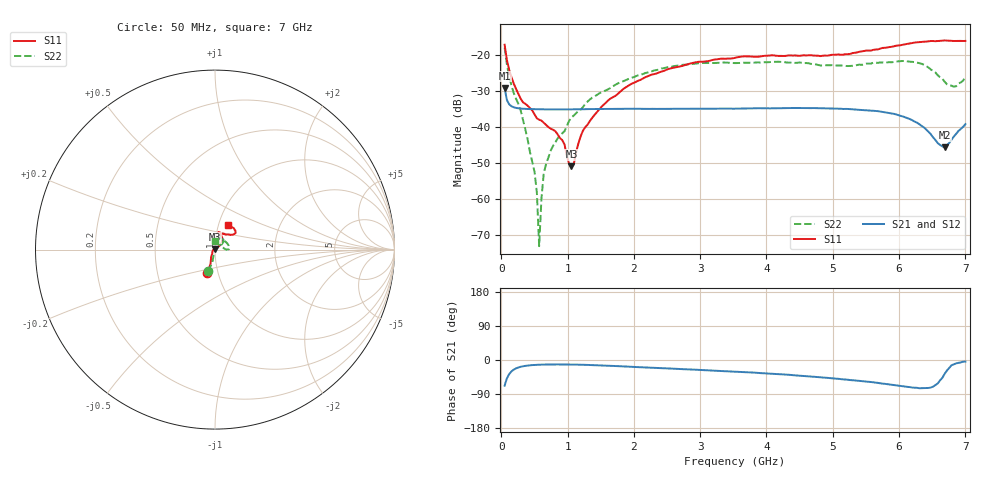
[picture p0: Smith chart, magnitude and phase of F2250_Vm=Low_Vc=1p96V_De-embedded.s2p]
! Integrated Device Technology
! Corporate Headquarters
! 6024 Silver Creek Valley Road
! San Jose, CA 95138  USA
! Phone:  1-408-284-8200
! Toll Free:  1-800-223-1366
! Webpage:  http://www.idt.com/
! Timing and RF Division
! 515 Groton Road, Suite 102
! Westford, MA 01886-6024
! Device:  F2250
! Description: Voltage Variable RF Attenuator
! Frequency:  50.0 -  6000.00 MHz
! Package:  3x3 mm Thin QFN Plastic Package: 16 pin
! Ports:  2 RF, 3 DC
!  Pin  1  = GND
!  Pin  2  = NC
!  Pin  3  = RF1  = Port 1
!  Pin  4  = NC
!  Pin  5  = GND
!  Pin  6  = GND
!  Pin  7  = GND
!  Pin  8  = GND
!  Pin  9  = NC
!  Pin 10  = RF2  = Port 2
!  Pin 11  = NC
!  Pin 12  = GND
!  Pin 13  = GND
!  Pin 14  = VCNTRL
!  Pin 15  = VDD
!  Pin 16  = VMODE
! Vcntrl:  1.960 Volts
! Vmode:  +0.000 Volts
! Vdd:  +3.30  Volts
! Current:  1.182 mA
! Data:  The device was measured on a the F2250 evaluation board which has
!  individual transmission lines to the RF pins.  Data was collected
!  using a calibrated network analyzer.  The evaluation board was
!  de-embedded using a TRL calibration technique.
!  The reference plane is the edge of the package pin.
! Misc:  SN 10
!  Action Tracker AT0258
! Date Measured:  2014-11-26
! Date:  2015-10-15  MJV
! Note:
!  Integrated Device Technology supplies this data as a sample of measured
!  data at the package pin for this product.  Your particular data for this
!  product may vary.
!  Data was taken at 25 degrees C.
!  Integrated Device Technology reserves the right to change this data at anytime.
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# GHz S dB R 50
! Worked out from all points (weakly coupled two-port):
!   201 points, 50 MHz to 7 GHz, reference 50 ohm
!   highest |S21| = -29.22 dB at 50 MHz (marker M1); lowest = -45.7 dB at 6.687 GHz (marker M2)
!   lowest |S11| = -51.0 dB at 1.058 GHz (marker M3), VSWR 1.01, Z = 49.9 + j0.24 ohm
!   |S11| at or under -10 dB: start of sweep to end of sweep
!   |S22| runs from -73.1 to -18.0 dB; largest |S21 - S12| = 5.4e-05
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0.05  -17.18 -108.6  -29.22 -67.7  -29.22 -67.7  -17.97 -107.5
0.08475  -21.44 -107.4  -32.55 -48.5  -32.55 -48.4  -22.72 -101.4
0.189  -28.01 -119.5  -34.55 -25.3  -34.55 -25.2  -30.64 -104.6
0.29325  -32.21 -127.5  -34.90 -17.9  -34.90 -17.9  -35.52 -100.5
0.50175  -36.50 -149.7  -35.08 -13.1  -35.08 -13.0  -52.55 -112.2
0.5365  -37.61 -155.2  -35.10 -12.7  -35.10 -12.7  -58.23 -112.2
0.57125  -37.99 -160.1  -35.11 -12.4  -35.11 -12.4  -73.12 -126.5
0.606  -38.25 -160.8  -35.12 -12.2  -35.12 -12.2  -59.76 49.3
0.64075  -38.86 -161.1  -35.12 -12.1  -35.12 -12.0  -52.87 50.5
0.6755  -39.50 -163.3  -35.13 -11.9  -35.13 -11.9  -50.28 49.0
0.91875  -43.67 157.8  -35.15 -11.7  -35.15 -11.7  -41.79 46.4
1.05775  -50.96 121.7  -35.13 -12.0  -35.14 -12.0  -37.41 47.5
1.2315  -41.04 43.7  -35.08 -12.6  -35.08 -12.6  -34.49 35.6
1.6485  -32.10 41.7  -35.01 -15.3  -35.01 -15.3  -29.16 39.0
2.37825  -24.87 47.3  -34.99 -21.2  -34.98 -21.2  -24.05 43.2
3.525  -20.81 72.4  -34.93 -30.8  -34.94 -30.8  -22.28 67.3
4.7065  -20.18 72.3  -34.77 -44.0  -34.77 -44.1  -22.57 68.0
5.85325  -17.82 40.4  -36.16 -64.5  -36.15 -64.5  -22.02 15.4
6.33975  -16.41 40.9  -39.73 -74.3  -39.73 -74.4  -22.47 1.3
6.68725  -15.99 48.8  -45.67 -36.4  -45.70 -36.0  -27.45 21.6
6.861  -16.13 55.1  -41.91 -8.9  -41.87 -8.9  -28.70 58.9
7  -16.12 63.2  -39.23 -4.2  -39.19 -4.3  -26.12 89.0
